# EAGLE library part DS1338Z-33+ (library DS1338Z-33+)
Real Time Clock Serial 56Byte Maxim DS1338Z-33+ Real Time Clock Battery Backup, Calendar, Clock, NV Timekeeping RAM, 56B RAM 8-Pin SOIC Source: Datasheet
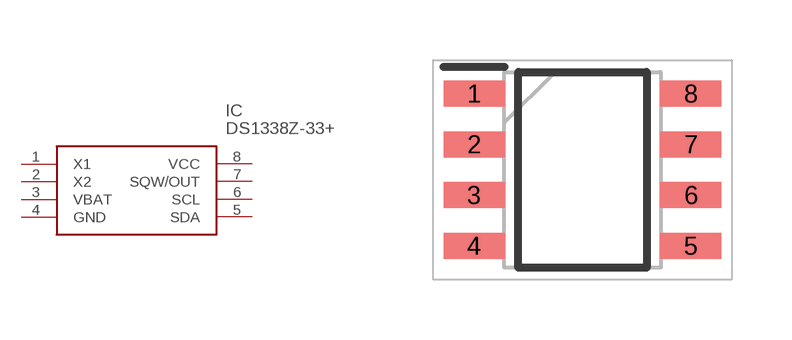
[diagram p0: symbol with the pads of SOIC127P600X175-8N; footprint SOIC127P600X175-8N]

Designator prefix IC

## DS1338Z-33+ (Arrow_Part_Number: DS1338Z-33+; Arrow_Price-Stock: https://www.arrow.com/en/products/ds1338z-33/maxim-integrated?region=europe; Description: Real Time Clock Serial 56Byte Maxim DS1338Z-33+ Real Time Clock Battery Backup, Calendar, Clock, NV Timekeeping RAM, 56B RAM 8-Pin SOIC; Height: 1.75mm; Manufacturer_Name: Analog Devices; Manufacturer_Part_Number: DS1338Z-33+; Mouser_Part_Number: 700-DS1338Z-33; Mouser_Price-Stock: https://www.mouser.co.uk/ProductDetail/Analog-Devices-Maxim-Integrated/DS1338Z-33%2b?qs=0Y9aZN%252BMVCVblIXsYVg1wg%3D%3D)  [SOIC127P600X175-8N]
1  X1
2  X2
3  VBAT
4  GND
5  SDA
6  SCL
7  SQW/OUT
8  VCC

## Footprint SOIC127P600X175-8N (pad centres in mm)
8 SO-3
smd 1.525 x 0.65: 1 -2.712,1.905; 2 -2.712,0.635; 3 -2.712,-0.635; 4 -2.712,-1.905; 5 2.712,-1.905; 6 2.712,-0.635; 7 2.712,0.635; 8 2.712,1.905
